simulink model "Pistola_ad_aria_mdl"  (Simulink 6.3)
settings: Solver=ode45  StartTime=0.0  StopTime=10.0  RelTol=1e-6
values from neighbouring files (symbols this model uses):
  A0 = 2*cm^2    (= 0.0002)    [Pistola_ad_aria.m]
  Ap = 0.3*cm^2    (= 3e-05)    [Pistola_ad_aria.m]
  b0 = 0.8*N/(10*cm/sec)    (= 8)    [Pistola_ad_aria.m]
  bp = 0.005*N/(10*cm/sec)    (= 0.05)    [Pistola_ad_aria.m]
  bt = bm+b1*(r0/r1)^2+b3*(r0*r2/(r1*r3))^2+b5*(r0*r2*r4/(r1*r3*r5))^2    (= 0.0109583333333)    [Pistola_ad_aria.m]
  Imax = 10000*Amp    (= 10000)    [Pistola_ad_aria.m]
  Jt = Jm+J1*(r0/r1)^2+J3*(r0*r2/(r1*r3))^2+J5*(r0*r2*r4/(r1*r3*r5))^2    (= 3.6984375e-05)    [Pistola_ad_aria.m]
  K0 = 1*200*N/(5*cm)    (= 4000)    [Pistola_ad_aria.m]
  K7 = 100*N/(1*mm)    (= 100000)    [Pistola_ad_aria.m]
  Ke = 0.5*N*m/Amp    (= 0.5)    [Pistola_ad_aria.m]
  La = 0.05*Henry    (= 0.05)    [Pistola_ad_aria.m]
  m0 = 50*gr    (= 0.05)    [Pistola_ad_aria.m]
  mp = 30*gr    (= 0.03)    [Pistola_ad_aria.m]
  P0 = 1*bar    (= 100000)    [Pistola_ad_aria.m]
  r6 = 3.5*r0    (= 0.035)    [Pistola_ad_aria.m]
  Ra = 2*Ohm    (= 2)    [Pistola_ad_aria.m]
  rt = r0*r2*r4/(r1*r3*r5)    (= 0.0416666666667)    [Pistola_ad_aria.m]
  Tau_r = 0*N*m    (= 0)    [Pistola_ad_aria.m]
  Tc = Tfin/8000    (= 0.000625)    [Pistola_ad_aria.m]
  Th3_0 = 0    [Pistola_ad_aria.m]
  V0 = pi*r6*A0    (= 2.19911485751e-05)    [Pistola_ad_aria.m]
  Va = 30*V    (= 30)    [Pistola_ad_aria.m]

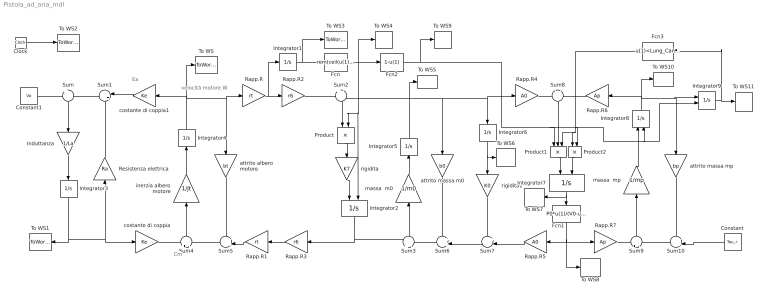
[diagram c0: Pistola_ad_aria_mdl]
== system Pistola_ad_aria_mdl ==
  note: Ea
  note: velocità motore W
  note: Cm
  Clock : Clock
  Constant : Constant  Orientation=left  Value=Tau_r
  Constant1 : Constant  Value=Va
  Fcn : Fcn  Expr=rem(ceil(u(1)/pi),2)
  Fcn1 : Fcn  Orientation=down  Expr=P0*u(1)/(V0-u(1))
  Fcn2 : Fcn  Expr=1-u(1)
  Fcn3 : Fcn  Orientation=left  Expr=u(1)<Lung_Canna
  Induttanza : Gain  Orientation=down  Gain=1/La
  Integrator1 : Integrator  InitialCondition=Th3_0
  Integrator2 : Integrator  Orientation=down  ExternalReset=falling
  Integrator3 : Integrator  Orientation=down  UpperSaturationLimit=Imax  LowerSaturationLimit=-Imax
  Integrator4 : Integrator  Orientation=up
  Integrator5 : Integrator  Orientation=up
  Integrator6 : Integrator  Orientation=down
  Integrator7 : Integrator  Orientation=down  ExternalReset=either
  Integrator8 : Integrator  Orientation=up  ExternalReset=rising
  Integrator9 : Integrator  ExternalReset=rising
  Product : Product  Orientation=down
  Product1 : Product  Orientation=down  Inputs=3
  Product2 : Product  Orientation=down
  Rapp.R : Gain  Gain=rt
  Rapp.R1 : Gain  Orientation=left  Gain=rt
  Rapp.R2 : Gain  Gain=r6
  Rapp.R3 : Gain  Orientation=left  Gain=r6
  Rapp.R4 : Gain  Gain=A0
  Rapp.R5 : Gain  Orientation=left  Gain=A0
  Rapp.R6 : Gain  Orientation=left  Gain=Ap
  Rapp.R7 : Gain  Gain=Ap
  Resistenza elettrica : Gain  Orientation=up  Gain=Ra
  Sum : Sum  Orientation=down  Inputs=+|-
  Sum1 : Sum  Orientation=left  Inputs=|++
  Sum10 : Sum  Orientation=left  Inputs=++|
  Sum2 : Sum  Orientation=down  Inputs=+|-
  Sum3 : Sum  Orientation=up  Inputs=+|-
  Sum4 : Sum  Orientation=up  Inputs=+|-
  Sum5 : Sum  Orientation=left  Inputs=++|
  Sum6 : Sum  Orientation=left  Inputs=++|
  Sum7 : Sum  Orientation=left  Inputs=+-|
  Sum8 : Sum  Orientation=down  Inputs=-|-
  Sum9 : Sum  Orientation=up  Inputs=+|-
  To WS : ToWorkspace  VariableName=Wm  SampleTime=Tc  SaveFormat=Array
  To WS1 : ToWorkspace  VariableName=Ia  SampleTime=Tc  SaveFormat=Array
  To WS10 : ToWorkspace  VariableName=Xpdot  SampleTime=Tc  SaveFormat=Array
  To WS11 : ToWorkspace  VariableName=Xp  SampleTime=Tc  SaveFormat=Array
  To WS2 : ToWorkspace  VariableName=t  SampleTime=Tc  SaveFormat=Array
  To WS3 : ToWorkspace  VariableName=Th3  SampleTime=Tc  SaveFormat=Array
  To WS4 : ToWorkspace  VariableName=Car  SampleTime=Tc  SaveFormat=Array
  To WS5 : ToWorkspace  VariableName=X0dot  SampleTime=Tc  SaveFormat=Array
  To WS6 : ToWorkspace  VariableName=X0  SampleTime=Tc  SaveFormat=Array
  To WS7 : ToWorkspace  VariableName=Vx  SampleTime=Tc  SaveFormat=Array
  To WS8 : ToWorkspace  VariableName=Px  SampleTime=Tc  SaveFormat=Array
  To WS9 : ToWorkspace  VariableName=Scar  SampleTime=Tc  SaveFormat=Array
  attrito albero motore : Gain  Orientation=down  Gain=bt
  attrito massa m0 : Gain  Orientation=down  Gain=b0
  attrito massa mp : Gain  Orientation=down  Gain=bp
  costante di coppia : Gain  Gain=Ke
  costante di coppia1 : Gain  Orientation=left  Gain=Ke
  inerzia albero motore : Gain  Orientation=up  Gain=1/Jt
  massa  m0 : Gain  Orientation=up  Gain=1/m0
  massa  mp : Gain  Orientation=up  Gain=1/mp
  rigidita : Gain  Orientation=down  Gain=K7
  rigidita1 : Gain  Orientation=down  Gain=K0
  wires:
  Clock/1 -> To WS2/1
  Sum/1 -> Induttanza/1
  Induttanza/1 -> Integrator3/1
  Sum1/1 -> Sum/2
  Resistenza elettrica/1 -> Sum1/2
  Sum4/1 -> inerzia albero motore/1
  inerzia albero motore/1 -> Integrator4/1
  Sum5/1 -> Sum4/2
  attrito albero motore/1 -> Sum5/1
  Integrator4/1 -> costante di coppia1/1, To WS/1, attrito albero motore/1, Rapp.R/1
  costante di coppia1/1 -> Sum1/1
  costante di coppia/1 -> Sum4/1
  Integrator3/1 -> Resistenza elettrica/1, costante di coppia/1, To WS1/1
  Constant1/1 -> Sum/1
  Rapp.R1/1 -> Sum5/2
  Rapp.R/1 -> Rapp.R2/1, Integrator1/1
  Rapp.R3/1 -> Rapp.R1/1
  Integrator1/1 -> To WS3/1, Fcn/1
  rigidita/1 -> Integrator2/1
  Rapp.R2/1 -> Sum2/1
  Integrator2/1 -> Rapp.R3/1, Sum3/1
  Fcn/1 -> To WS4/1, Product/2, Integrator2/2, Fcn2/1
  Sum2/1 -> Product/1
  Product/1 -> rigidita/1
  Sum3/1 -> massa  m0/1
  massa  m0/1 -> Integrator5/1
  Sum6/1 -> Sum3/2
  attrito massa m0/1 -> Sum6/1
  Integrator5/1 -> Sum2/2, To WS5/1, attrito massa m0/1, Integrator6/1, Rapp.R4/1
  Integrator6/1 -> rigidita1/1, To WS6/1
  rigidita1/1 -> Sum7/1
  Sum7/1 -> Sum6/2
  Rapp.R5/1 -> Sum7/2
  Integrator7/1 -> To WS7/1, Fcn1/1
  Rapp.R4/1 -> Sum8/1
  Rapp.R6/1 -> Sum8/2
  Sum9/1 -> massa  mp/1
  massa  mp/1 -> Integrator8/1
  Sum10/1 -> Sum9/2
  attrito massa mp/1 -> Sum10/1
  Rapp.R7/1 -> Sum9/1
  Integrator8/1 -> Rapp.R6/1, To WS10/1, attrito massa mp/1, Integrator9/1
  Constant/1 -> Sum10/2
  Fcn2/1 -> To WS9/1, Product1/1, Integrator8/2, Integrator9/2, Product2/2
  Fcn1/1 -> Rapp.R5/1, Rapp.R7/1, To WS8/1
  Integrator9/1 -> To WS11/1, Fcn3/1
  Product1/1 -> Integrator7/1
  Sum8/1 -> Product1/2
  Product2/1 -> Integrator7/2
  Fcn3/1 -> Product2/1, Product1/3
